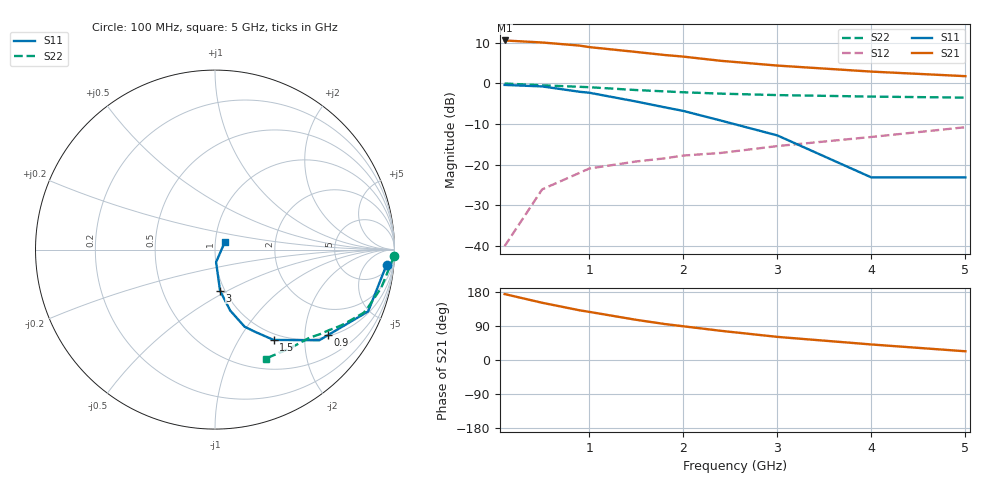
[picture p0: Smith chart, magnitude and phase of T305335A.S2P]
!AT-30533
!S and NOISE PARAMETERS at Vce=5V  Ic=1mA.  LAST UPDATED 06-23-94
# ghz s ma r 50!
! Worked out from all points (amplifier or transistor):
!   11 points, 100 MHz to 5 GHz, reference 50 ohm
!   highest |S21| = 10.6 dB at 100 MHz (marker M1)
!   |S21| within 3 dB of that: start of sweep to 1.568 GHz
!   unconditionally stable (mu >= 1): 2.645 GHz to 4.366 GHz
!   at 500 MHz: K = 0.28, MSG = 18.0 dB, |S12| = -26.0 dB
!   at 1.8 GHz: K = 0.80, MSG = 12.7 dB, |S12| = -18.4 dB
!   at 5 GHz: K = 0.95, MSG = 6.3 dB, |S12| = -10.8 dB
!   lowest NFmin = 0.30 dB at 500 MHz
!   S11 on the Smith chart (normalised r, x): 100 MHz: 9, -19; 900 MHz: 1.04, -2.62; 1.5 GHz: 0.91, -1.42; 3 GHz: 0.95, -0.46; 5 GHz: 1.11, +0.10
0.1  0.96 -5.0  3.38 174.0  0.01 85.0  0.999 -2.0
0.5  0.92 -22.0  3.19 151.0  0.05 74.0  0.95 -13.0
0.9  0.79 -37.0  2.92 131.0  0.08 65.0  0.91 -21.0
1  0.77 -41.0  2.8 127.0  0.09 63.0  0.9 -23.0
1.5  0.6 -57.0  2.44 106.0  0.11 56.0  0.83 -30.0
1.8  0.51 -64.0  2.24 95.0  0.12 54.0  0.8 -33.0
2  0.46 -69.0  2.14 89.0  0.13 52.0  0.78 -35.0
2.4  0.35 -76.0  1.9 77.0  0.14 51.0  0.75 -39.0
3  0.23 -83.0  1.66 61.0  0.17 51.0  0.72 -43.0
4  0.07 -85.0  1.4 41.0  0.22 52.0  0.69 -53.0
5  0.07 38.0  1.23 23.0  0.29 49.0  0.67 -65.0
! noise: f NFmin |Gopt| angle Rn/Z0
0.5  0.3  0.94  7  1.02
0.9  0.4  0.89  16  0.98
1.8  0.9  0.75  43  0.58
2.4  1.3  0.65  65  0.38
